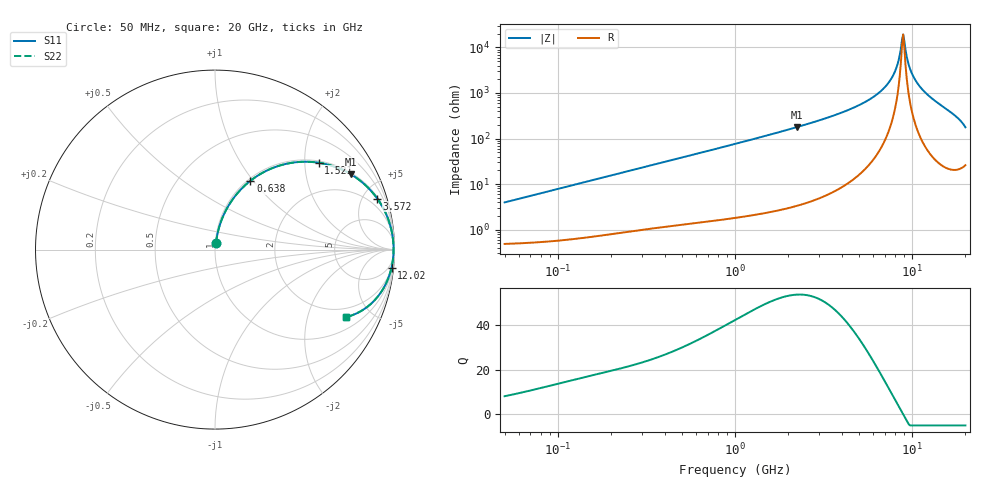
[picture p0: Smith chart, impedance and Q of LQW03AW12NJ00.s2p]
!Murata Part Number: LQW03AW12NJ00
!These Parameters are Measured in Series Mode Connection
!  o--[Z]--o
!Port1  Port2
!  o-------o
!Freq. Start=50[MHz] Stop=20[GHz], 401[Steps]
# Hz S RI R 50
!Freq.(Hz) S11(Real) S11(Imag) S21(Real) S21(Imag) S12(Real) S12(Imag) S22(Real) S22(Imag)
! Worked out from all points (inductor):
!   401 points, 50 MHz to 20 GHz, reference 50 ohm
!   read as one part in series: L = 12.4 nH near 51.52 MHz
!   highest Q = 53.6 at 2.245 GHz (marker M1), where L = 12.7 nH
!   self-resonance near 8.775 GHz
!   S11 on the Smith chart (normalised r, x): 50 MHz: 1.01, +0.08; 638 MHz: 1.03, +0.97; 1.521 GHz: 1.05, +2.34; 3.572 GHz: 1.13, +6.31; 12.02 GHz: 2, -19; 20 GHz: 1.52, -3.50
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5e7  0.00631 0.0387  0.9937 -0.0387  0.9937 -0.0387  0.00631 0.0387
1.364002e8  0.0173 0.1034  0.9827 -0.1034  0.9827 -0.1034  0.0173 0.1034
3.721004e8  0.0831 0.2573  0.9169 -0.2573  0.9169 -0.2573  0.0831 0.2573
6.380365e8  0.1968 0.3831  0.8032 -0.3831  0.8032 -0.3831  0.1968 0.3831
1e9  0.3692 0.4709  0.6308 -0.4709  0.6308 -0.4709  0.3692 0.4709
1.521052e9  0.5768 0.4841  0.4232 -0.4841  0.4232 -0.4841  0.5768 0.4841
2.245319e9  0.7572 0.4195  0.2428 -0.4195  0.2428 -0.4195  0.7572 0.4195
2.728004e9  0.8289 0.3672  0.1711 -0.3672  0.1711 -0.3672  0.8289 0.3672
3.572216e9  0.9037 0.2846  0.0963 -0.2846  0.0963 -0.2846  0.9037 0.2846
5.683258e9  0.9752 0.1381  0.0248 -0.1381  0.0248 -0.1381  0.9752 0.1381
6.601595e9  0.9864 0.092  0.0136 -0.092  0.0136 -0.092  0.9864 0.092
7.442007e9  0.9919 0.0553  0.00809 -0.0553  0.00809 -0.0553  0.9919 0.0553
8.141811e9  0.9942 0.0277  0.00582 -0.0277  0.00582 -0.0277  0.9942 0.0277
8.644534e9  0.9948 0.00907  0.00519 -0.00907  0.00519 -0.00907  0.9948 0.00907
8.907419e9  0.9949 -0.000302  0.00515 0.000302  0.00515 0.000302  0.9949 -0.000302
9.041845e9  0.9948 -0.00501  0.0052 0.00501  0.0052 0.00501  0.9948 -0.00501
9.600142e9  0.9941 -0.024  0.00588 0.024  0.00588 0.024  0.9941 -0.024
1.004137e10  0.9931 -0.0386  0.00691 0.0386  0.00691 0.0386  0.9931 -0.0386
1.082228e10  0.9903 -0.0634  0.00975 0.0634  0.00975 0.0634  0.9903 -0.0634
1.201863e10  0.9835 -0.0999  0.0165 0.0999  0.0165 0.0999  0.9835 -0.0999
1.696185e10  0.9118 -0.2559  0.0882 0.2559  0.0882 0.2559  0.9118 -0.2559
2e10  0.7286 -0.3767  0.2714 0.3767  0.2714 0.3767  0.7286 -0.3767
